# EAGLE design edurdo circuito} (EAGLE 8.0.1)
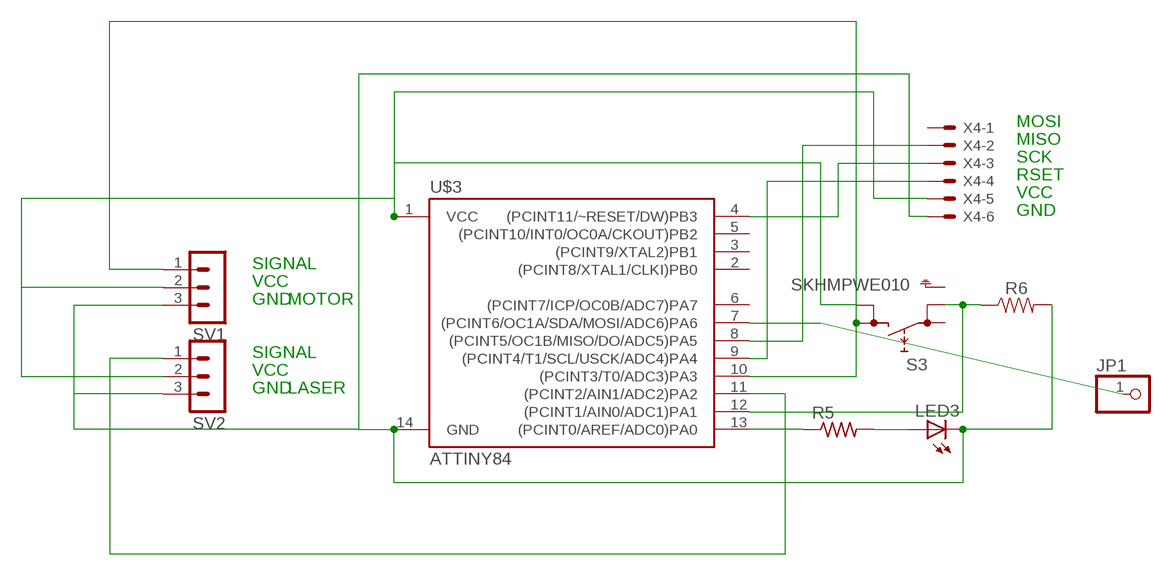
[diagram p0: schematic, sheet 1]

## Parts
JP1  PINHD-1X1  [1X01]
LED3  LED1206  [LED-1206]
R5  R-US_R1206  [R1206]
R6  RESISTOR1206  [1206]
S3  SKHMPWE010  [SKHMPXE010]
SV1  MA03-1  [MA03-1]
SV2  MA03-1  [MA03-1]
U$3  ATTINY84  [SO14]
X4  22-23-2061  [22-23-2061]

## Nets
N$12: S3.3(2.1) SV1.1 U$3.10((PCINT3/T0/ADC3)PA3)
N$13: SV2.1 U$3.11((PCINT2/AIN1/ADC2)PA2)
N$17: R5.1 U$3.13((PCINT0/AREF/ADC0)PA0)
N$18: LED3.A R5.2
N$19: LED3.C R6.2 SV1.3 SV2.3 U$3.14(GND) X4.6
N$20: R6.1 S3.2(1.2) U$3.12((PCINT1/AIN0/ADC1)PA1)
N$22: S3.4(2.2) SV1.2 SV2.2 U$3.1(VCC) X4.5
N$23: U$3.4((PCINT11/~RESET/DW)PB3) X4.4
N$24: U$3.8((PCINT5/OC1B/MISO/DO/ADC5)PA5) X4.2
N$25: JP1.1 U$3.7((PCINT6/OC1A/SDA/MOSI/ADC6)PA6)
N$26: U$3.9((PCINT4/T1/SCL/USCK/ADC4)PA4) X4.3
Unconnected: S3.1(1.1) S3.5(SH) U$3.2((PCINT8/XTAL1/CLKI)PB0) U$3.3((PCINT9/XTAL2)PB1) U$3.5((PCINT10/INT0/OC0A/CKOUT)PB2) U$3.6((PCINT7/ICP/OC0B/ADC7)PA7) X4.1

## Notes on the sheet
- MOSI
- MISO
- SCK
- RSET
- VCC
- GND
- SIGNAL
- VCC
- GND | MOTOR
- SIGNAL
- VCC
- GND | LASER

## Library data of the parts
JP1 = pinhead:PINHD-1X1: PIN HEADER
LED3 = SparkFun-Retired:LED: LEDs
R5 = resistor:R-US_: RESISTOR, American symbol
R6 = SparkFun-Resistors:RESISTOR: Generic Resistor Package
S3 = switch:SKHMP*E010: 6.2 X 6.5mm TACT Switch (SMD) Source: http://www3.alps.co.jp/WebObjects/catalog.woa/PDF/E/Switch/Tact/SKHM/SKHM.PDF
SV1 SV2 = con-lstb:MA03-1: PIN HEADER; OC_FARNELL: unknown; OC_NEWARK: unknown
U$3 = SparkFun-IC-Microcontroller:ATTINY84: Atmel 14-pin 2/4/8kB flash uC Datasheet SparkFun Products Tiny AVR Programmer (PGM-11801) SparkFun Servo Trigger - Continuous Rotation (WIG-13872) SparkFun Servo Trigger (WIG-13118); PROD_ID: IC-11285
X4 = con-molex:22-23-2061: .100" (2.54mm) Center Header - 6 Pin; MF: MOLEX; MPN: 22-23-2061; OC_FARNELL: 1462922; OC_NEWARK: 27C1933

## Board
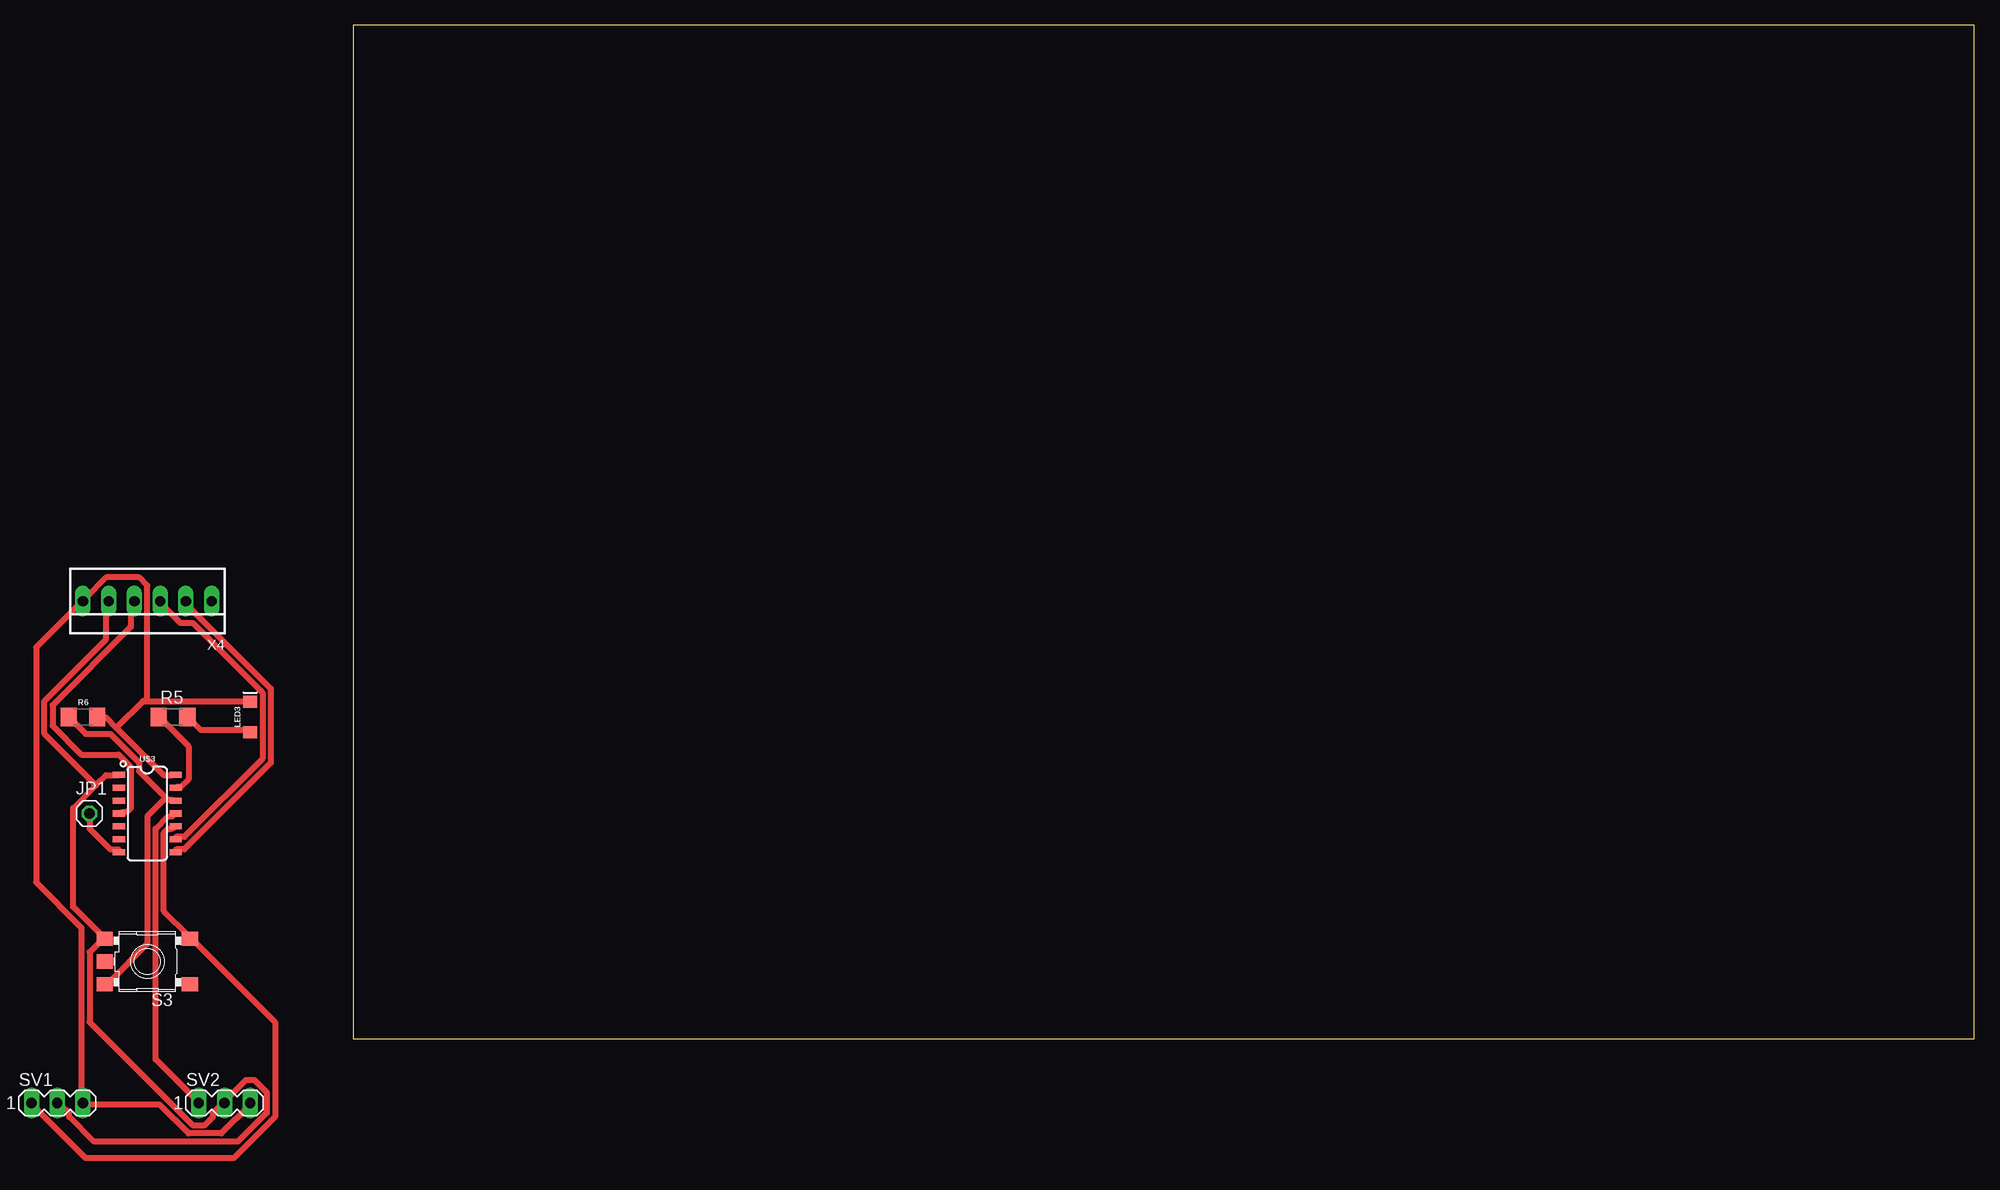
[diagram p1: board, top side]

Size 160 x 100 mm. Coordinates in mm from the lower left corner, seen from the top.
Outline: 0,0 160,0 160,100 0,100 0,0
Copper layers (1*16): Top 0.035mm / dielectric 1.5mm / Bottom 0.035mm
Design rules "default *": minimum track width 24mil, minimum drill 24mil, track to track 10mil, track to pad 12mil, pad to pad 12mil, via to via 12mil, smd to smd 8mil, copper to edge 40mil, drill to drill 8mil, minimum pad ring 10mil, minimum via ring 8mil, stop-mask expansion 4mil, vias tented up to drill 0mil, thermal gap 10mil

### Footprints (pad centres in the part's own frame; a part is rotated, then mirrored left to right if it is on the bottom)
1X01 = drill 1.016 octagon: 1 0,0
LED-1206 = smd 1.2 x 1.4: A -1.5,0; C 1.5,0
R1206 = smd 1.6 x 1.803: 1 -1.422,0; 2 1.422,0
1206 = smd 1.6 x 1.8: 1 -1.4,0; 2 1.4,0
SKHMPXE010 = smd 1.6 x 1.4: 1 -4.2,2.25; 2 4.2,2.25; 3 -4.2,-2.25; 4 4.2,-2.25; 5 4.2,0
MA03-1 = drill 1.016 long: 1 -2.54,0; 2 0,0; 3 2.54,0
SO14 = smd 0.6 x 1.2: 1 -3.175,-2.8; 2 -1.905,-2.8; 3 -0.635,-2.8; 4 0.635,-2.8; 5 1.905,-2.8; 6 3.175,-2.8; 7 4.445,-2.8; 8 4.445,2.8; 9 3.175,2.8; 10 1.905,2.8; 11 0.635,2.8; 12 -0.635,2.8; 13 -1.905,2.8; 14 -3.175,2.8
22-23-2061 = drill 1 long: 1 -6.35,0; 2 -3.81,0; 3 -1.27,0; 4 1.27,0; 5 3.81,0; 6 6.35,0

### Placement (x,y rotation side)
JP1  -26.04,22.23 0 top  (outside the outline)
LED3  -10.16,31.75 90 top  (outside the outline)
R5  -17.78,31.75 0 top  (outside the outline)
R6  -26.67,31.75 0 top  (outside the outline)
S3  -20.32,7.62 180 top  (outside the outline)
SV1  -29.21,-6.35 0 top  (outside the outline)
SV2  -12.7,-6.35 0 top  (outside the outline)
U$3  -20.32,22.86 270 top  (outside the outline)
X4  -20.32,43.18 180 top  (outside the outline)

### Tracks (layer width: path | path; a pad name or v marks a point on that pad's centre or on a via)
N$12
  Top 0.61: U$3.10 -17.88,20.73 -18.29,20.73 -18.69,20.32 -18.69,12.6 -16.26,10.16 S3.3 -15.85,9.75 -7.72,1.63 -7.72,-7.72 -11.79,-11.79 -26.42,-11.79 -31.7,-6.5 SV1.1
N$13
  Top 0.61: U$3.11 -17.88,21.95 -18.29,21.95 -19.51,20.73 -19.51,-2.03 -15.44,-6.1 SV2.1
N$17
  Top 0.61: U$3.13 -17.48,24.79 -17.07,24.79 -16.26,25.6 -16.26,28.85 -19.1,31.7 R5.1
N$18
  Top 0.61: LED3.A -10.16,30.48 -15.04,30.48 -16.26,31.7 R5.2
N$19
  Top 0.61: SV2.3 -10.16,-6.5 -13.01,-9.35 -16.26,-9.35 -19.1,-6.5 -26.42,-6.5 SV1.3 -26.82,-6.1 -26.82,10.97 -31.29,15.44 -31.29,38.61 -26.82,43.08 X4.6 -26.42,43.48 -24.38,45.52 -21.13,45.52 -20.32,44.7 -20.32,33.33 | -23.37,30.68 -24.38,31.7 -25.2,31.7 R6.2 | -23.37,30.68 -18.69,26.01 -17.88,26.01 U$3.14 | -20.32,33.33 -20.73,33.33 -23.37,30.68 | -20.32,33.33 -10.16,33.33 LED3.C
N$20
  Top 0.61: -18.49,23.77 -21.13,26.42 -21.13,27.23 -23.98,30.07 -26.42,30.07 -28.04,31.7 R6.1 | -18.49,23.77 -18.29,23.57 -17.88,23.57 U$3.12 | -18.49,23.77 -20.32,21.95 -20.32,9.35 -23.98,5.69 -24.38,5.69 S3.2
N$22
  Top 0.61: SV1.2 -28.85,-6.5 -28.04,-7.32 -28.04,-7.72 -25.6,-10.16 -11.38,-10.16 -8.53,-7.32 -8.53,-5.28 -9.75,-4.06 -10.57,-4.06 -12.6,-6.1 SV2.2 -13.01,-6.5 -13.82,-7.32 -13.82,-7.72 -14.63,-8.53 -15.85,-8.53 -26.01,1.63 -26.01,8.53 -24.79,9.75 S3.4 -24.79,10.16 -27.64,13.01 -27.64,22.76 -25.4,24.99 | -25.4,24.99 -24.38,26.01 -23.16,26.01 U$3.1 | -25.4,24.99 -30.48,30.07 -30.48,33.33 -24.38,39.42 -24.38,43.08 X4.5
N$23
  Top 0.61: U$3.4 -22.76,22.35 -22.35,22.35 -21.95,22.76 -21.95,26.82 -23.16,28.04 -26.82,28.04 -29.67,30.89 -29.67,32.92 -21.95,40.64 -21.95,43.08 X4.4
N$24
  Top 0.61: U$3.8 -17.48,18.69 -16.66,18.69 -8.13,27.23 -8.13,34.54 -16.66,43.08 X4.2
N$25
  Top 0.61: U$3.7 -23.16,18.69 -23.98,18.69 -26.01,20.73 -26.01,21.95 JP1.1
N$26
  Top 0.61: U$3.9 -17.48,19.91 -16.66,19.91 -8.94,27.64 -8.94,34.14 -15.85,41.05 -17.07,41.05 -19.1,43.08 X4.3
